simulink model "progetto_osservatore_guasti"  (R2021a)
settings: Solver=VariableStepAuto  StartTime=0.0  StopTime=10  RelTol=1e-3
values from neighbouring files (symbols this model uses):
  A = [0.9944 -0.1203 -0.4302    [esempio_progetto_oss_SISO.m]
  Ao = A - K*C    [esempio_progetto_oss_SISO.m]
  B = [0.4252 -0.0082 0.1813]'    [esempio_progetto_oss_SISO.m]
  Bo = [B K]    [esempio_progetto_oss_SISO.m]
  C = [1 0 0]    [esempio_progetto_oss_SISO.m]
  Co = C    [esempio_progetto_oss_SISO.m]
  D = zeros(m,r)    [esempio_progetto_oss_SISO.m]
  Do = zeros(m,r+m)    [esempio_progetto_oss_SISO.m]
  Tc = 0.1    [esempio_progetto_oss_SISO.m]
  x0 = 0.05    [esempio_progetto_oss_SISO.m]

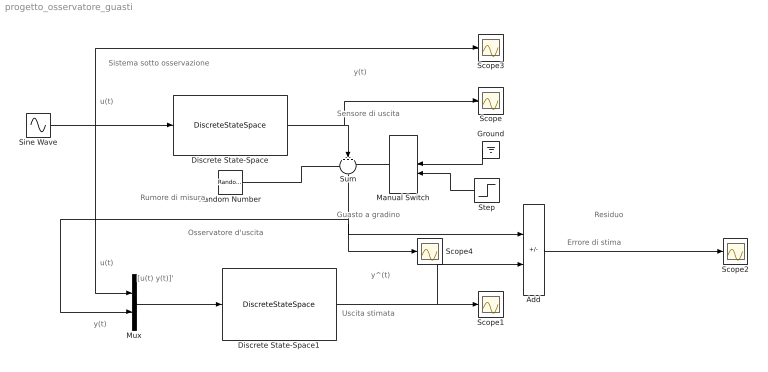
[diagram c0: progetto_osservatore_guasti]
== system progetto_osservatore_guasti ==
  note: Guasto a gradino
  note: Rumore di misura
  note: Sensore di uscita
  note: Residuo
  note: Errore di stima
  note: y^(t)
  note: Uscita stimata
  note: [u(t) y(t)]'
  note: y(t)
  note: u(t)
  note: Osservatore d'uscita
  note: Sistema sotto osservazione
  note: y(t)
  note: u(t)
  Add : Sum  Inputs=+-
  Discrete State-Space : DiscreteStateSpace  A=A  B=B  C=C  D=D  InitialCondition=x0  SampleTime=Tc
  Discrete State-Space1 : DiscreteStateSpace  A=Ao  B=Bo  C=Co  D=Do  SampleTime=Tc
  Ground : Ground
  Manual Switch : ManualSwitch  CurrentSetting=0
  Mux : Mux  Inputs=2
  Random Number : RandomNumber  Variance=(0.0002)^2  SampleTime=0.01
  Scope{,1..4} (5 alike) : Scope
  Sine Wave : Sin  SampleTime=0
  Step : Step  Time=5  After=100  SampleTime=0
  Sum : Sum  Inputs=+++
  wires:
  Sine Wave/1 -> Scope3/1, Mux/1, Discrete State-Space/1
  Discrete State-Space/1 -> Scope/1, Sum/2
  Mux/1 -> Discrete State-Space1/1
  Discrete State-Space1/1 -> Add/2, Scope1/1
  Add/1 -> Scope2/1
  Sum/1 -> Scope4/1, Add/1, Mux/2
  Ground/1 -> Manual Switch/1
  Step/1 -> Manual Switch/2
  Manual Switch/1 -> Sum/3
  Random Number/1 -> Sum/1
